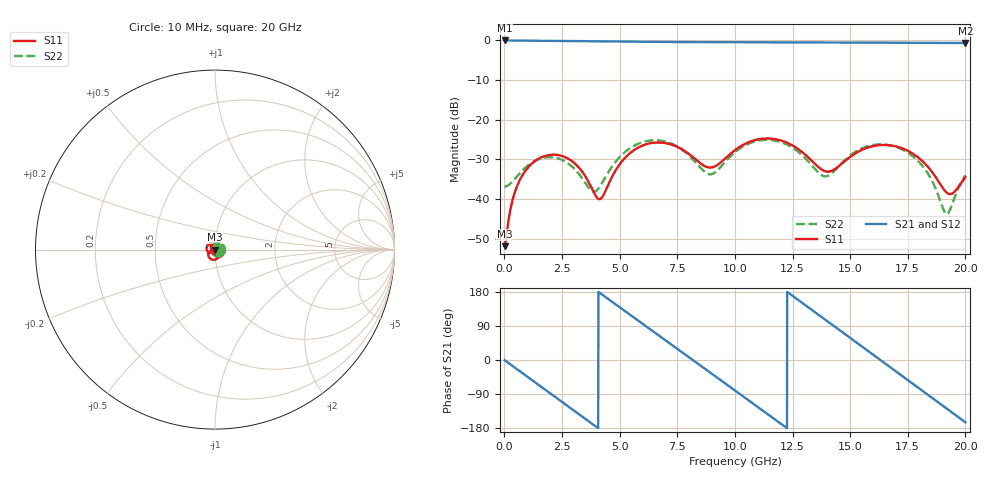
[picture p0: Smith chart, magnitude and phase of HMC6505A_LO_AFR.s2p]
! Analog Devices, Inc.
! 1 Analog Way
! Wilmington, MA 01887
! http://www.analog.com
! Date:  2021-09-17 NN
! Board Name:  EV1HMC6505ALC5 (125487-1) with HMC6505ALC5 installed
! File Description:  Automatic Fixture Removal S-Parameters for LO Port connector and board loss de-embedding
! File Generation:  Calibrated Network Analyzer
! Chip Part Number:  HMC6505A
! Chip Description:  GaAs, MMIC, IQ Upconverter
! Chip Frequency:  5.5 to 8.6 GHz
! Chip Package:  LCC, 4.9 x 4.9 x 1 mm
! LO Port:  HMC6505ALC5 removed and end of trace left open
! Note:
!  Analog Devices supplies this data as a sample of measured data at the evaluation board
!  ports for this product.  Your particular data for this product may vary.
!  Analog Devices reserves the right to change this data at anytime.
!  All lines below in this file are as is from the Network Analyzer.
!Agilent Technologies,N5245A,MY52451809,A.10.47.06
!Automatic Fixture Removal (AFR)
!Date: Friday, September 17, 2021 3:14:08 AM
!S2P File: Measurements: S11,S21,S12,S22:
# MHz S  RI  R 50
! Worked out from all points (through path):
!   2000 points, 10 MHz to 20 GHz, reference 50 ohm
!   highest |S21| = 0.00 dB at 10 MHz (marker M1); lowest = -0.6 dB at 20 GHz (marker M2)
!   group delay of S21, straight-line fit = 123 ps
!   lowest |S11| = -51.9 dB at 10 MHz (marker M3), VSWR 1.01, Z = 49.7 + j0.0287 ohm
!   |S11| at or under -10 dB: start of sweep to end of sweep
!   |S22| runs from -43.8 to -25.1 dB; largest |S21 - S12| = 1.5e-15
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10  -0.00252 0.000288  0.9998 -0.00774  0.9998 -0.00774  0.0143 0.000137
630  0.00569 0.0154  0.8797 -0.4665  0.8797 -0.4665  0.0194 0.00661
1770  0.0339 0.0085  0.1983 -0.9682  0.1983 -0.9682  0.0327 -0.00626
2520  0.033 -0.0105  -0.3618 -0.9148  -0.3618 -0.9148  0.0223 -0.0214
3350  0.0161 -0.0158  -0.832 -0.5156  -0.832 -0.5156  -0.00208 -0.0185
4110  0.00956 -0.00264  -0.9735 0.029  -0.9735 0.029  -0.0127 0.0056
4730  0.0192 0.0072  -0.8481 0.4699  -0.8481 0.4699  -0.00178 0.027
5740  0.0431 -0.00459  -0.2763 0.9219  -0.2763 0.9219  0.0392 0.029
6680  0.0393 -0.0334  0.3968 0.8713  0.3968 0.8713  0.054 -0.0096
8300  0.00469 -0.0312  0.9488 -0.0912  0.9488 -0.0912  -0.00887 -0.0274
8990  0.00947 -0.0231  0.7719 -0.557  0.7719 -0.557  -0.0203 0.00328
10010  0.0193 -0.0366  0.1534 -0.9374  0.1534 -0.9374  0.011 0.0374
10860  0.00357 -0.0551  -0.4473 -0.836  -0.4473 -0.836  0.0477 0.0233
11830  -0.0287 -0.0483  -0.8949 -0.3093  -0.8949 -0.3093  0.0498 -0.0206
13340  -0.0286 -0.00981  -0.6354 0.7003  -0.6354 0.7003  -0.0114 -0.0238
13980  -0.0194 -0.0107  -0.2253 0.9172  -0.2253 0.9172  -0.019 0.00372
14810  -0.0241 -0.0191  0.3697 0.8669  0.3697 0.8669  0.00202 0.0317
15790  -0.0442 -0.00735  0.8629 0.372  0.8629 0.372  0.0394 0.0247
16670  -0.0424 0.022  0.9017 -0.2558  0.9017 -0.2558  0.0474 -0.00605
18320  0.0021 0.0264  0.00943 -0.9334  0.00943 -0.9334  0.00371 -0.0218
19180  0.000309 0.0121  -0.5713 -0.7351  -0.5713 -0.7351  -0.00643 0.000254
20000  -0.00854 0.0168  -0.8944 -0.2476  -0.8944 -0.2476  0.00538 0.0191
